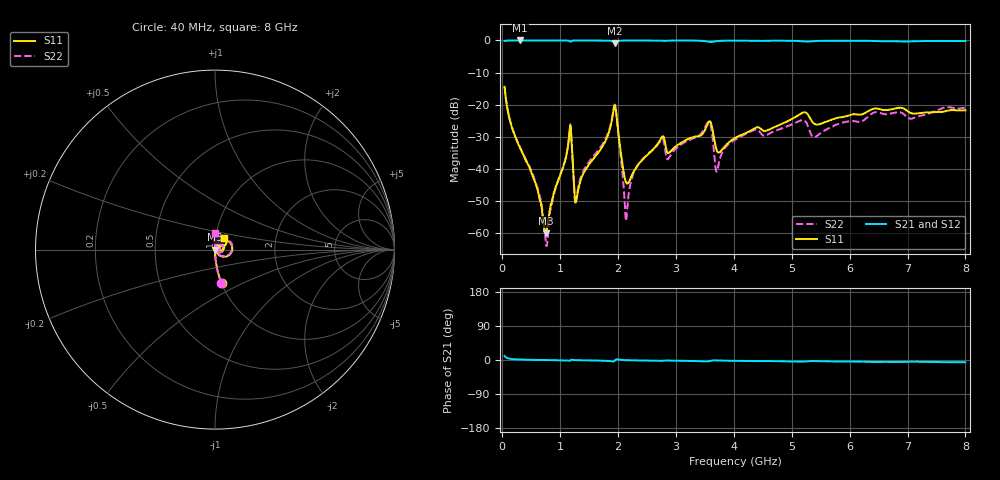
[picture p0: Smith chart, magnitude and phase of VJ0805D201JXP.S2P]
! VJ0805D201JXP
! DATE 03/14/2022  09:03
! CAPACITORS MOUNTED IN SERIES ON 25 MIL THICK MICROSTRIP SUBSTRATE
# GHz  S  MA  R  50.00
!  FREQ  S11M  S11A  S21M  S21A  S12M  S12A  S22M  S22A
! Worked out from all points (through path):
!   801 points, 40 MHz to 8 GHz, reference 50 ohm
!   highest |S21| = 0.00 dB at 308.6 MHz (marker M1); lowest = -0.9 dB at 1.95 GHz (marker M2)
!   lowest |S11| = -60.1 dB at 756.4 MHz (marker M3), VSWR 1.00, Z = 50.1 + j0.0158 ohm
!   |S11| at or under -10 dB: start of sweep to end of sweep
!   |S22| runs from -64.1 to -14.4 dB; largest |S21 - S12| = 0.0033
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0.04  0.1891 -78.9  0.9816 10.9  0.9808 10.9  0.1914 -79.2
0.14945  0.04983 -86.9  0.9982 2.8  0.9984 2.8  0.05014 -86.9
0.30865  0.02093 -88.1  0.9997 1.2  0.9994 1.1  0.02167 -88.0
0.60715  0.004765 -83.2  0.9994 0.2  0.9992 0.2  0.005062 -83.6
0.7564  0.0009897 9.2  0.9991 -0.1  0.9994 -0.2  0.0006497 -10.8
1.1544  0.03203 56.8  0.9844 -1.9  0.9846 -1.9  0.03325 62.5
1.1942  0.02946 -35.9  0.9754 0.7  0.9756 0.7  0.03029 -30.9
1.2738  0.003123 20.9  0.9976 -0.4  0.9978 -0.4  0.003034 36.4
1.3733  0.007385 69.3  0.9984 -0.7  0.9989 -0.8  0.008137 80.3
1.7713  0.02595 72.9  0.9952 -1.9  0.995 -1.9  0.02775 83.0
1.9504  0.09657 -4.1  0.9032 -0.4  0.9034 -0.4  0.09781 1.3
2.13945  0.006112 -12.6  0.9962 -0.5  0.9965 -0.5  0.001532 18.9
2.3086  0.01023 51.5  0.9975 -1.1  0.998 -1.1  0.01021 92.0
2.69665  0.02522 57.5  0.9935 -2.0  0.9941 -2.1  0.02441 85.8
2.87575  0.01764 38.9  0.9933 -1.5  0.9937 -1.5  0.0147 77.7
3.5623  0.05321 33.3  0.9541 -3.4  0.9537 -3.4  0.05356 52.5
3.71155  0.01879 9.8  0.9806 -1.1  0.9808 -1.1  0.009353 63.1
4.02995  0.03049 52.6  0.9926 -2.3  0.9927 -2.4  0.02875 94.4
5.1742  0.07364 44.1  0.9719 -4.3  0.972 -4.3  0.05714 76.9
5.3533  0.05413 25.8  0.9716 -2.7  0.9719 -2.7  0.03206 66.4
6.67665  0.08308 51.1  0.9741 -5.1  0.9743 -5.2  0.07152 80.3
8  0.08169 52.0  0.9799 -5.9  0.9803 -6.0  0.08993 91.4
